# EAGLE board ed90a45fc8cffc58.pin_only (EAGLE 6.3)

Size 60 x 60 mm. Coordinates in mm from the lower left corner, seen from the top.
Outline: 0,0 60,0 60,60 0,60 0,0
Copper layers (1*16): Top 0.035mm / dielectric 1.5mm / Bottom 0.035mm
Design rules "adafruit *": minimum track width 8mil, minimum drill 15.5mil, track to track 8mil, track to pad 8mil, pad to pad 8mil, via to via 8mil, smd to smd 8mil, copper to edge 10mil, drill to drill 8mil, minimum pad ring 10mil, minimum via ring 8mil, stop-mask expansion 4mil, vias tented up to drill 20mil, thermal gap 10mil

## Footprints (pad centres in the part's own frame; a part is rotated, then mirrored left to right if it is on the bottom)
SOLDERJUMPER_REFLOW_NOPASTE = smd 1.168 x 1.6: 1 -0.762,0; 2 0.762,0
_0805 = smd 1.2 x 1.3: 1 -1.016,0; 2 1.016,0
SOD-323 = smd 1.35 x 0.8: A 1.27,0; C -1.27,0
SOD-323F = smd 1 x 0.8: A -1,0; C 1,0
FIDUCIAL_1MM = smd 1 x 1: 1 0,0
1X5_SMT = smd 1.27 x 5.08: 1 -5.08,0; 2 -2.54,0; 3 0,0; 4 2.54,0; 5 5.08,0
LED3MM-4X4GRID = drill 0.813 pad 1.524 octagon: A1 -21.23,-22.5; A2 -6.23,-22.5; A3 8.77,-22.5; A4 23.77,-22.5; A5 -21.23,-7.5; A6 -6.23,-7.5; A7 8.77,-7.5; A8 23.77,-7.5; A9 -21.23,7.5; A10 -6.23,7.5; A11 8.77,7.5; A12 23.77,7.5; A13 -21.23,22.5; A14 -6.23,22.5; A15 8.77,22.5; A16 23.77,22.5; K1 -23.77,-22.5; K2 -8.77,-22.5; K3 6.23,-22.5; K4 21.23,-22.5; K5 -23.77,-7.5; K6 -8.77,-7.5; K7 6.23,-7.5; K8 21.23,-7.5; K9 -23.77,7.5; K10 -8.77,7.5; K11 6.23,7.5; K12 21.23,7.5; K13 -23.77,22.5; K14 -8.77,22.5; K15 6.23,22.5; K16 21.23,22.5
R0805 = smd 1.3 x 1.5: 1 -0.95,0; 2 0.95,0
ELAST_PAD_SQUARE_10MM_5.4MM_4X4GRID = smd 0.4 x 0.4: A1 -17.5,-22.5; A2 -2.5,-22.5; A3 12.5,-22.5; A4 27.5,-22.5; A5 -17.5,-7.5; A6 -2.5,-7.5; A7 12.5,-7.5; A8 27.5,-7.5; A9 -17.5,7.5; A10 -2.5,7.5; A11 12.5,7.5; A12 27.5,7.5; A13 -17.5,22.5; A14 -2.5,22.5; A15 12.5,22.5; A16 27.5,22.5 | smd 0.4 x 2: B1 -27.33,-22.51; B2 -12.33,-22.51; B3 2.67,-22.51; B4 17.67,-22.51; B5 -27.33,-7.51; B6 -12.33,-7.51; B7 2.67,-7.51; B8 17.67,-7.51; B9 -27.33,7.49; B10 -12.33,7.49; B11 2.67,7.49; B12 17.67,7.49; B13 -27.33,22.49; B14 -12.33,22.49; B15 2.67,22.49; B16 17.67,22.49 | hole 2.8: -28,-15; -2,-15; 28,-15; -28,15; -2,15; 2,15; 28,15; 2,-15 | hole 1: -28.7,-28.7; 28.7,-28.7; 28.7,28.7; -28.7,28.7 | hole 2: -15,15; 15,15; 15,-15; -15,-15
TESTPOINT_SMT = smd 4.7 x 3.4: P$1 0,0
SOP28_300MIL = smd 0.635 x 2.286: P$1 -8.255,-5.08; P$2 -6.985,-5.08; P$3 -5.715,-5.08; P$4 -4.445,-5.08; P$5 -3.175,-5.08; P$6 -1.905,-5.08; P$7 -0.635,-5.08; P$8 0.635,-5.08; P$9 1.905,-5.08; P$10 3.175,-5.08; P$11 4.445,-5.08; P$12 5.715,-5.08; P$13 6.985,-5.08; P$14 8.255,-5.08; P$15 8.255,5.08; P$16 6.985,5.08; P$17 5.715,5.08; P$18 4.445,5.08; P$19 3.175,5.08; P$20 1.905,5.08; P$21 0.635,5.08; P$22 -0.635,5.08; P$23 -1.905,5.08; P$24 -3.175,5.08; P$25 -4.445,5.08; P$26 -5.715,5.08; P$27 -6.985,5.08; P$28 -8.255,5.08
MOUNTINGHOLE_2.5_PLATED = drill 2.5 pad 3.2: P$1 0,0

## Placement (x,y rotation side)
A0  [SOLDERJUMPER_REFLOW_NOPASTE]  42.67,20.32 180 bottom
A1  [SOLDERJUMPER_REFLOW_NOPASTE]  35.05,20.32 180 bottom
A2  [SOLDERJUMPER_REFLOW_NOPASTE]  49.78,20.32 180 bottom
C1  [_0805]  6.35,28.7 270 bottom
C2  [_0805]  53.59,28.7 270 bottom
C3  [_0805]  28.45,6.6 0 bottom
C4  [_0805]  28.7,53.34 0 bottom
C5  10uF  [_0805]  40.89,33.53 90 bottom
D1  1N4148  [SOD-323]  40.42,13.67 0 bottom
D2  1N4148  [SOD-323]  45.46,36.29 90 bottom
D4  1N4148  [SOD-323F]  36.32,16 0 bottom
D5  1N4148  [SOD-323]  51.31,33.78 270 bottom
D6  1N4148  [SOD-323]  20.83,16.26 180 bottom
D7  1N4148  [SOD-323]  20.57,13.46 0 bottom
D8  1N4148  [SOD-323]  38.1,47.24 180 bottom
D9  1N4148  [SOD-323]  38.1,45.47 180 bottom
D10  1N4148  [SOD-323]  39.88,11.43 180 bottom
D11  1N4148  [SOD-323]  35.05,11.43 180 bottom
D12  1N4148  [SOD-323]  48.77,45.72 0 bottom
D13  1N4148  [SOD-323]  26.92,20.83 270 bottom
FID1  FIDUCIAL""  [FIDUCIAL_1MM]  54.1,3.05 0 bottom
FID2  FIDUCIAL""  [FIDUCIAL_1MM]  1.52,11.68 0 bottom
FID3  FIDUCIAL""  [FIDUCIAL_1MM]  47.5,50.8 0 bottom
JP1  [1X5_SMT]  57.4,29.97 90 bottom
JP2  [1X5_SMT]  2.54,29.97 90 bottom
JP3  [1X5_SMT]  29.97,2.54 180 bottom
JP4  [1X5_SMT]  29.97,57.4 180 bottom
LED1  TBD  [LED3MM-4X4GRID]  30,30 180 top
R1  10K  [_0805]  33.27,39.37 180 bottom
R2  10K  [_0805]  39.12,39.37 0 bottom
R3  47K  [R0805]  35.05,18.03 180 bottom
R4  47K  [R0805]  42.67,18.03 0 bottom
R5  47K  [R0805]  49.53,18.03 180 bottom
SW1  [ELAST_PAD_SQUARE_10MM_5.4MM_4X4GRID]  30,30 180 top
TP1  [TESTPOINT_SMT]  1.52,29.97 90 top
TP2  [TESTPOINT_SMT]  30.23,1.52 0 top
TP3  [TESTPOINT_SMT]  29.97,58.42 0 top
TP4  [TESTPOINT_SMT]  58.42,29.97 90 top
U1  HT16K33 28SOP  [SOP28_300MIL]  30,30 0 bottom
U$1  MOUNTINGHOLE2.5  [MOUNTINGHOLE_2.5_PLATED]  14.99,29.97 0 top
U$2  MOUNTINGHOLE2.5  [MOUNTINGHOLE_2.5_PLATED]  44.96,29.97 0 top
U$3  [ADAFRUIT_TEXT_20MM]  21.72,0.38 0 bottom

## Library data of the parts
A0 A1 A2 C1-C5 D1 D2 D5-D13 JP1-JP4 LED1 R1 R2 SW1 TP1-TP4 U1 U$3 = microbuilder
D4 = adafruit
FID1-FID3 U$1 U$2 = microbuilder; BOM: EXCLUDE
R3-R5 = rcl

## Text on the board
tPlace: All 3mm LEDs have Anode on left side! | 1 | 2 | 3 | 4 | 5 | 6 | 7 | 8 | 9 | 10 | 11 | 12 | 13 | 15 | 16 | 14 | All 3mm LEDs have Anode on left side!
bPlace: SDA | INT | SCL | 5V | GND | Adafruit Trellis | 4x4 Elastomer / Buttons+LEDs | SDA | SDA | SCL | SCL | GND | GND | 5V | 5V | INT | INT | A1 | A0 | A2 | Up to 8 can / be tiled when | 5V | GND | SCL | addrs are unique | INT | SDA

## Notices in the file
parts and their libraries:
microbuilder: This work is placed in the public domain, and may be freely used for commercial and non-commercial work with the following conditions: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
